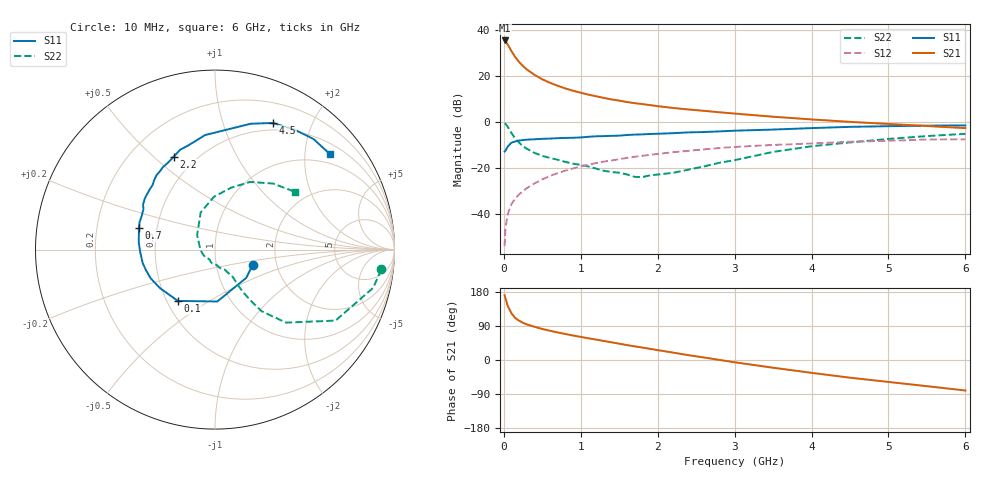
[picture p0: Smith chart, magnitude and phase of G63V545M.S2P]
! SIEMENS Small Signal Semiconductors
! BFG193
! Si NPN RF Bipolar Junction Transistor in SOT223
! VCE = 3.5 V  IC = 45 mA
! Common Emitter S-Parameters:  August  1996
# GHz  S  MA  R  50
!  f  S11  S21  S12  S22
! GHz  MAG  ANG  MAG  ANG  MAG  ANG  MAG  ANG
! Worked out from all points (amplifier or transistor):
!   36 points, 10 MHz to 6 GHz, reference 50 ohm
!   highest |S21| = 35.3 dB at 10 MHz (marker M1)
!   |S21| within 3 dB of that: start of sweep to 71.63 MHz
!   unconditionally stable (mu >= 1): 452.4 MHz to 2.358 GHz
!   at 250 MHz: K = 0.91, MSG = 27.1 dB, |S12| = -30.1 dB
!   at 1.4 GHz: K = 1.04, MAG = 11.9 dB, |S12| = -16.8 dB
!   at 6 GHz: K = 0.90, MSG = 2.4 dB, |S12| = -7.6 dB
!   S11 on the Smith chart (normalised r, x): 10 MHz: 1.50, -0.27; 100 MHz: 0.57, -0.37; 700 MHz: 0.39, +0.12; 2.2 GHz: 0.38, +0.58; 4.5 GHz: 0.42, +1.48; 6 GHz: 0.74, +2.58
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0.01  0.2265 -22.1  58.14 171.1  0.002 90.1  0.9327 -6.8
0.02  0.2347 -42.1  56.26 163.6  0.0047 80.1  0.9067 -13.6
0.05  0.2894 -87.4  47.65 142.9  0.0099 71.4  0.7793 -30.5
0.1  0.353 -125.9  33.97 122.9  0.0165 66.5  0.5675 -45.8
0.15  0.3746 -145.2  25.01 110.5  0.0217 65.1  0.4301 -52.9
0.2  0.3921 -155.7  19.75 103.5  0.0267 66.7  0.3514 -54.9
0.25  0.4016 -163.5  16.11 98.0  0.0313 67.6  0.294 -56.3
0.3  0.4099 -169.6  13.62 93.8  0.0364 68.7  0.26 -56.9
0.4  0.417 -178.1  10.4 87.7  0.0461 68.5  0.2108 -57.1
0.5  0.4268 174.5  8.35 81.8  0.0563 67.9  0.1817 -57.0
0.6  0.4318 169.3  7.011 77.2  0.0668 67.0  0.1645 -58.2
0.7  0.441 164.2  6.043 72.7  0.0768 66.1  0.15 -60.4
0.9  0.4497 155.3  4.716 64.6  0.0974 62.1  0.1233 -64.2
1.1  0.4732 147.9  3.881 57.3  0.1169 58.6  0.1071 -74.5
1.3  0.4881 141.1  3.296 50.2  0.1367 54.5  0.0864 -84.2
1.6  0.516 130.9  2.683 39.3  0.1647 47.7  0.0721 -109.2
2.2  0.5656 114.1  1.994 19.5  0.2185 34.3  0.0779 -173.8
2.8  0.6186 99.3  1.609 0.3  0.2697 20.3  0.1288 140.7
3.5  0.6775 83.0  1.288 -20.4  0.3144 3.0  0.2219 111.1
4.5  0.7759 65.4  0.995 -46.7  0.3683 -17.0  0.3566 75.4
5.5  0.825 48.3  0.809 -69.1  0.4123 -40.2  0.4894 48.8
6  0.8325 39.8  0.729 -80.5  0.4179 -53.7  0.5488 36.0
